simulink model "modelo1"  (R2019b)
settings: Solver=ode45  StartTime=0.0  StopTime=100  RelTol=1e-3  EnableMultiTasking=on
undefined symbols (not defined in the file): Kc, magnitude, Ti
libraries: simulink x1

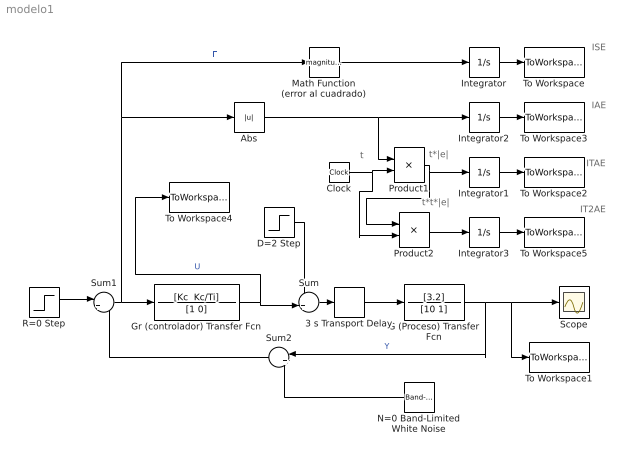
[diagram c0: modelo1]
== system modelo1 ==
  note: t
  note: t*|e|
  note: IT2AE
  note: ITAE
  note: IAE
  note: ISE
  note: t*t*|e|
  3 s Transport Delay : TransportDelay  DelayTime=3
  Abs : Abs
  Clock : Clock
  D=2 Step : Step  Time=0  After=2  SampleTime=0
  G (Proceso) Transfer Fcn : TransferFcn  Numerator=[3.2]  Denominator=[10 1]
  Gr (controlador) Transfer Fcn : TransferFcn  Numerator="[Kc  Kc/Ti]"  Denominator=[1 0]
  Integrator{,1..3} (4 alike) : Integrator
  Math Function (error al cuadrado) : Math  Operator=magnitude^2
  N=0 Band-Limited White Noise : simulink/Sources/Band-Limited White Noise  Cov=[0.0]  Ts=0.1  seed=[23341]
  Product1 : Product
  Product2 : Product
  R=0 Step : Step  Time=0  After=0  SampleTime=0
  Scope : Scope
  Sum : Sum  Inputs=++|
  Sum1 : Sum  Inputs=|+-
  Sum2 : Sum  Inputs=|++
  To Workspace : ToWorkspace  VariableName=J1  SampleTime=-1
  To Workspace1 : ToWorkspace  VariableName=Y  SaveFormat=Timeseries  SampleTime=-1
  To Workspace2 : ToWorkspace  VariableName=J3  SampleTime=-1
  To Workspace3 : ToWorkspace  VariableName=J2  SampleTime=-1
  To Workspace4 : ToWorkspace  VariableName=U  SaveFormat=Timeseries  SampleTime=-1
  To Workspace5 : ToWorkspace  VariableName=J4  SampleTime=-1
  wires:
  Gr (controlador) Transfer Fcn/1 -> To Workspace4/1, Sum/2  "U"
  Sum1/1 -> Math Function (error al cuadrado)/1, Abs/1, Gr (controlador) Transfer Fcn/1  "E"
  R=0 Step/1 -> Sum1/1
  D=2 Step/1 -> Sum/1
  Sum2/1 -> Sum1/2
  G (Proceso) Transfer Fcn/1 -> To Workspace1/1, Scope/1, Sum2/1  "Y"
  3 s Transport Delay/1 -> G (Proceso) Transfer Fcn/1
  Sum/1 -> 3 s Transport Delay/1
  Math Function (error al cuadrado)/1 -> Integrator/1
  Integrator/1 -> To Workspace/1
  Clock/1 -> Product2/2, Product1/2
  Product1/1 -> Product2/1, Integrator1/1
  Integrator1/1 -> To Workspace2/1
  Integrator2/1 -> To Workspace3/1
  Abs/1 -> Product1/1, Integrator2/1
  Integrator3/1 -> To Workspace5/1
  Product2/1 -> Integrator3/1
  N=0 Band-Limited White Noise/1 -> Sum2/2
